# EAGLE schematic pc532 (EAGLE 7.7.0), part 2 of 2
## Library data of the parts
C1-C46 C48-C58 C61-C66 C69-C80 = alan_common:C_US: MLCC Ceramic cap
C47 C59 C60 C67 C68 = alan_common:C_POL_US
CONN1 CONN16 = alan_common:HDR_2X25: Centronics part TE 1734099-5
CONN2 = pc532:HDR_2X4
CONN3-CONN10 = alan_common:HDR_2X5: 0.254mm (100 mil) breakaway header - 2 x 5
CONN11 = alan_common:AT_POWER: IBM P8/P9 Style Motherboard Connector Pair
CONN12-CONN15 = pc532:ISA_SLOT8
D1-D3 = alan_common:D
F1 F2 = pc532:FUSE
J1 J2 = alan_common:HDR_1X3
J3 = alan_common:HDR_1X2: 1x2 100 mil jumper header
LED1-LED4 = pc532:LED_JUMPER
R1-R7 = alan_common:R_US
RES1 = alan_common:RNET_X5
RES2-RES11 RES15 RES16 = pc532:RA_SIP_X4
RES12 RES14 RES17 RES18 = pc532:SCSITERM
RES13 = alan_common:RNET_X15
SPARE1 = pc532:SPARE18
SPARE2 SPARE3 = pc532:SPARE20
SPARE4 = pc532:SPARE16
U1-U4 = pc532:74280
U5 U17 U21 U22 = alan_common:7404
U6-U13 = alan_common:SIMM_30: 30-pin SIMM Memory
U14 U15 = pc532:74832
U16 = alan_common:74374: Octal Edge Triggered Latch
U18 U23 U45 = alan_common:7407D
U19 U20 = alan_common:22V10
U24 = pc532:32381
U25 U34 = alan_common:XTAL_CAN_HALFSIZE
U26 U50 = alan_common:74174: Hex D-Latch
U27-U29 = pc532:74258
U30 = alan_common:7400
U31 U32 = alan_common:7474: Dual positive edge-triggered flip-flop with preset and clear
U33 = alan_common:74138
U35 = pc532:32532
U36 = pc532:746311
U37-U40 = alan_common:16V8: Atmel 16V8 Simple PLD
U41 = pc532:AIC6250
U42 = pc532:7414
U43 = alan_common:74646
U44 = alan_common:27C256
U46 = pc532:32202
U47 U49 U51 U53 U54 U56 U59 U61 = pc532:MC145406
U48 U52 U55 U60 = alan_common:SIGNETICS_SCN2681: Dual UART
U57 = pc532:DP8490
U58 = alan_common:7432
X1 = pc532:XTAL

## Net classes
0 default: width 0.203 mm, drill 0.33 mm, clearance 0.203 mm
1 power: width 0.813 mm, drill 0.33 mm, clearance 0.203 mm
